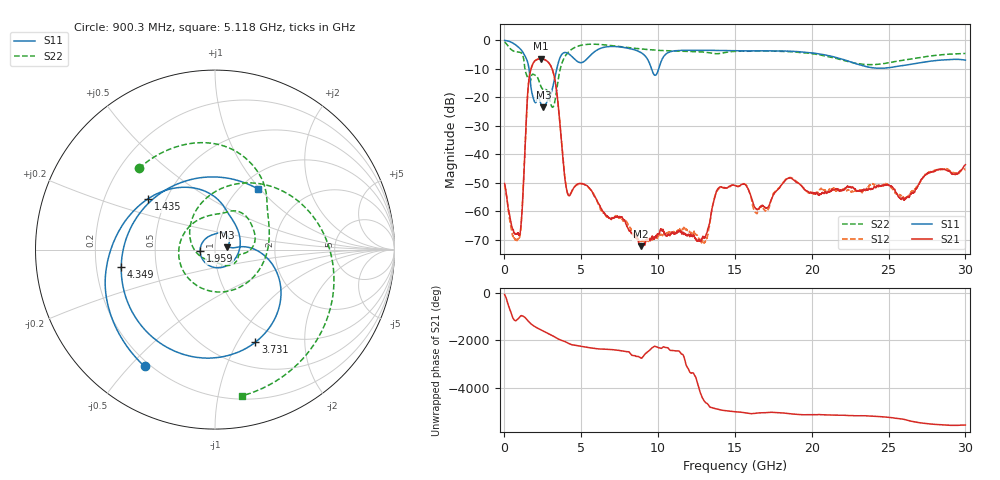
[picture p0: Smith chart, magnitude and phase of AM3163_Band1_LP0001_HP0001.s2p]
!Agilent Technologies,E8364B,MY43040894,A.07.50.67
!Agilent E8364B: A.07.50.67
!Date: Thursday, August 20, 2020 11:16:53
!Correction: S11(Full 2 Port(1,2))
!S21(Full 2 Port(1,2))
!S12(Full 2 Port(1,2))
!S22(Full 2 Port(1,2))
!S2P File: Measurements: S11, S21, S12, S22:
# Hz S  dB  R 50
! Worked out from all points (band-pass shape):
!   3201 points, 10 MHz to 30 GHz, reference 50 ohm
!   highest |S21| = -6.48 dB at 2.353 GHz (marker M1); lowest = -72.2 dB at 8.866 GHz (marker M2)
!   |S21| within 3 dB of the highest: 1.763 GHz to 3.058 GHz (1.295 GHz wide, 53.7 % of centre)
!   lowest |S11| = -23.5 dB at 2.531 GHz (marker M3), VSWR 1.14, Z = 57 + j1.4 ohm
!   |S11| at or under -10 dB: 1.597 GHz to 3.407 GHz (1.81 GHz wide, 72.3 % of centre); 9.568 GHz to 10.04 GHz (470.6 MHz wide, 4.8 % of centre)
!   |S22| runs from -23.5 to -0.6 dB; largest |S21 - S12| = 0.0049
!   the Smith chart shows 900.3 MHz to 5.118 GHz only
!   S11 on the Smith chart (normalised r, x): 900.3 MHz: 0.18, -0.55; 1.435 GHz: 0.40, +0.29; 1.959 GHz: 0.85, -0.01; 3.731 GHz: 0.79, -1.19; 4.349 GHz: 0.31, -0.08; 5.118 GHz: 1.20, +0.98
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1e7  -0.08 -8.8  -50.26 -84.7  -50.78 15.4  -0.63 -28.4
4.5985e8  -0.75 -60.5  -64.93 -178.0  -66.72 32.3  -3.38 -147.6
9.003281e8  -2.38 -121.1  -67.55 -13.7  -69.31 -68.9  -4.15 133.0
1.434525e9  -6.59 142.8  -26.03 -26.6  -25.99 -27.5  -12.14 -64.0
1.95935e9  -21.58 -175.0  -7.36 26.0  -7.35 26.0  -12.18 34.1
2.352969e9  -22.12 17.8  -6.48 -111.0  -6.48 -111.0  -15.94 -8.0
2.531034e9  -23.46 10.5  -6.63 -166.1  -6.63 -166.2  -17.33 -12.7
3.233925e9  -14.27 3.3  -12.55 -39.3  -12.57 -39.3  -22.53 -134.3
3.730634e9  -5.00 -66.4  -36.64 163.5  -36.55 163.9  -8.21 70.9
4.349178e9  -5.50 -169.7  -53.28 -9.6  -53.35 -10.4  -3.29 -14.4
5.014581e9  -7.85 73.3  -50.34 -85.5  -50.29 -85.9  -1.74 -72.1
5.117672e9  -7.66 54.3  -50.42 -96.0  -50.39 -96.4  -1.63 -79.6
6.373503e9  -2.62 -101.0  -59.77 161.4  -60.24 154.9  -1.56 -154.0
7.460641e9  -2.33 -173.7  -61.99 105.6  -62.20 102.4  -2.19 156.8
8.866422e9  -4.27 111.1  -72.24 152.4  -70.19 107.8  -3.04 101.2
1.000979e10  -10.49 115.8  -67.99 -134.1  -68.84 -84.6  -3.54 58.9
1.236213e10  -3.53 8.7  -68.86 152.9  -67.22 -145.7  -3.97 -21.6
1.5005e10  -3.65 -72.2  -51.01 68.3  -50.85 68.8  -3.91 -90.3
2.000958e10  -4.43 163.1  -53.43 -56.3  -53.74 -52.0  -4.71 136.7
2.275554e10  -8.03 60.1  -52.04 -98.9  -53.05 -96.8  -7.97 21.0
2.500479e10  -9.66 -62.2  -50.79 -165.2  -50.71 -166.1  -7.95 -91.9
3e10  -6.95 104.3  -43.65 -126.8  -45.42 -135.8  -4.64 102.3
